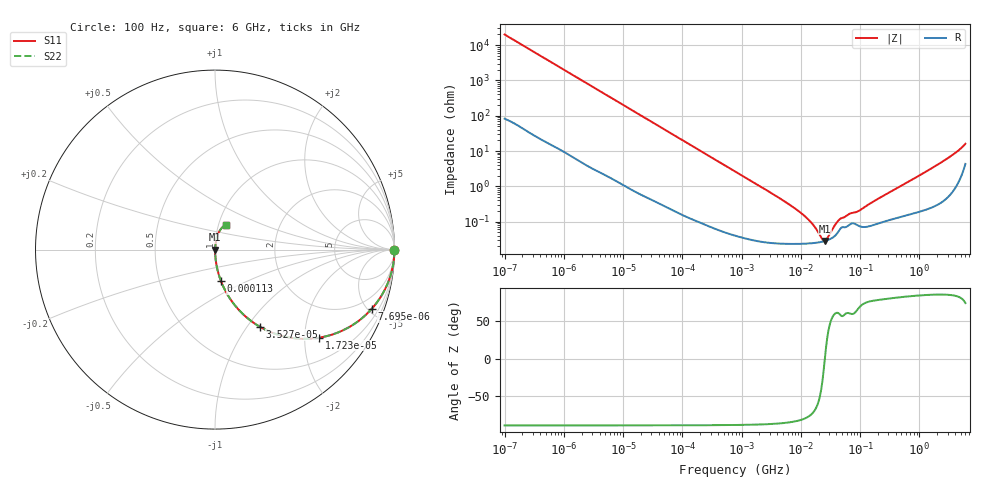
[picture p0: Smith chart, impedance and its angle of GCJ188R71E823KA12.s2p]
!Murata Part Number: GCJ188R71E823KA12
!These Parameters are Measured in Series Mode Connection
!Data Generated on Mar 13, 2026
!  o--ll--o
!Port1  Port2
!  o------o
!Operation Temp=25[degC], DC Bias Voltage=0[V]
!Freq. Start=100[Hz] Stop=6[GHz] 401[Steps]
# Hz S RI R 50
!Freq.(Hz) S11(Real) S11(Imag) S21(Real) S21(Imag) S12(Real) S12(Imag) S22(Real) S22(Imag)
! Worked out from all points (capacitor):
!   401 points, 100 Hz to 6 GHz, reference 50 ohm
!   read as one part in series: C = 79.4 nF near 109 Hz
!   lowest |Z| = 28.2 mohm at 25.46 MHz (marker M1)
!   series resonance near 25.47 MHz, so ESL is about 490 pH
!   S11 on the Smith chart (normalised r, x): 100 Hz: open; 7.695 kHz: 1.03, -5.27; 17.23 kHz: 1.01, -2.36; 35.27 kHz: 1.01, -1.16; 113 kHz: 1.00, -0.36; 6 GHz: 1.09, +0.31
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100  1 -0.005  4.56e-05 0.005  4.56e-05 0.005  1 -0.005
2008  0.9898 -0.0984  0.0102 0.0984  0.0102 0.0984  0.9898 -0.0984
4496  0.952 -0.2113  0.048 0.2113  0.048 0.2113  0.952 -0.2113
7695  0.8728 -0.3306  0.1272 0.3306  0.1272 0.3306  0.8728 -0.3306
17227  0.5815 -0.4905  0.4185 0.4905  0.4185 0.4905  0.5815 -0.4905
35265  0.2517 -0.4308  0.7483 0.4308  0.7483 0.4308  0.2517 -0.4308
40335  0.2051 -0.4005  0.7949 0.4005  0.7949 0.4005  0.2051 -0.4005
63115  0.0965 -0.2918  0.9035 0.2918  0.9035 0.2918  0.0965 -0.2918
112960  0.0331 -0.175  0.9669 0.175  0.9669 0.175  0.0331 -0.175
774597  0.00111 -0.0266  0.9989 0.0266  0.9989 0.0266  0.00111 -0.0266
6644369  0.000243 -0.00292  0.9998 0.00292  0.9998 0.00292  0.000243 -0.00292
1.087309e7  0.000239 -0.00157  0.9998 0.00157  0.9998 0.00157  0.000239 -0.00157
1.555665e7  0.000246 -0.000844  0.9998 0.000844  0.9998 0.000844  0.000246 -0.000844
2.225763e7  0.000267 -0.000224  0.9997 0.000224  0.9997 0.000224  0.000267 -0.000224
2.545746e7  0.000282 -5e-07  0.9997 5e-07  0.9997 5e-07  0.000282 -5e-07
2.784235e7  0.000296 0.00015  0.9997 -0.00015  0.9997 -0.00015  0.000296 0.00015
3.80911e7  0.000404 0.000712  0.9996 -0.000712  0.9996 -0.000712  0.000404 0.000712
4.556224e7  0.000605 0.00102  0.9994 -0.00102  0.9994 -0.00102  0.000605 0.00102
9.753859e7  0.000749 0.00192  0.9993 -0.00192  0.9993 -0.00192  0.000749 0.00192
3.124326e8  0.00115 0.00661  0.9988 -0.00661  0.9988 -0.00661  0.00115 0.00661
2.240541e9  0.00531 0.0449  0.9947 -0.0449  0.9947 -0.0449  0.00531 0.0449
6e9  0.0621 0.1392  0.9379 -0.1392  0.9379 -0.1392  0.0621 0.1392
